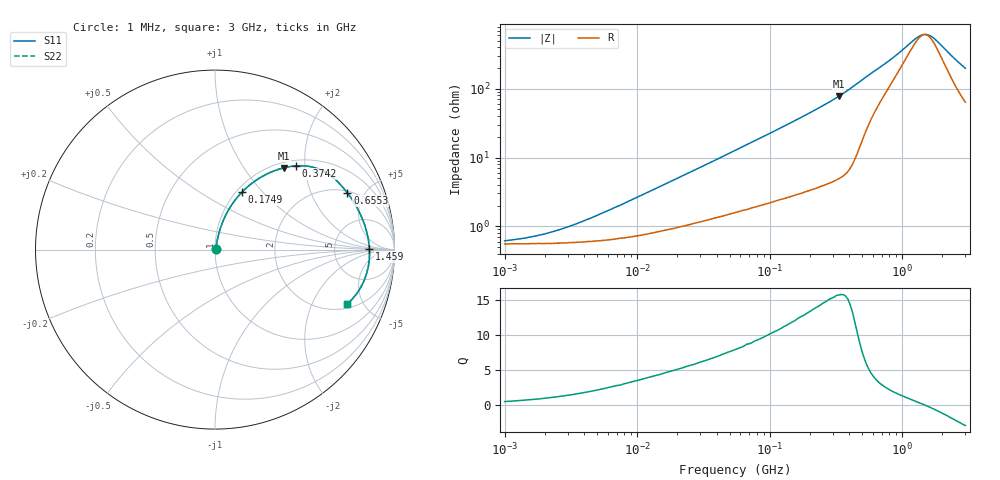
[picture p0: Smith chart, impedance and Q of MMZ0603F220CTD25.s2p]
! S-parameter Generated by TDK Corporation
! Copyright(C) 2018 TDK Corporation.
! All Rights Reserved.
! TDK P/N: MMZ0603F220CTD25 (Chip Bead)
! Property: |Z|=22¶ at 100MHz
! Size(LxWxT): 0.6x0.3x0.3mm, 0.024x0.012x0.012inches
! Model Type: s2p (Touchstone File Format Version 1.0)
! Frequency: DC=Yes Start=1MHz Stop=3000MHz 202points Log-sweep
! Model Generated on Aug. 6, 2018
! Port Assignments:
!  1 ---@@@--- 2
! Applicable Conditions:
!  Temperature = 25 degC
!  DC Bias Current = 0 A
!  Small Signal Operation
! Terms and conditions regarding TDK Simulation Models
! (1)This simulation model is being provided solely for informational purposes. Please refer to the specifications of the products in terms of detailed characteristics of such products.
! (2)In no event shall TDK Corporation of any of its subsidiaries be liable for any loss or damage arising, directly or indirectly,
!  From any information contained in this simulation model, including, but not limited to loss or damages arising from any inaccuracies, omissions or errors in connection with such information.
! (3)Any and all copyrights on this simulation model are owned by TDK Corporation.
!  Duplication or redistribution of this simulation model without prior written permission from TDK Corporation is prohibited.
! (4)This simulation model is subject to any modification or change without any prior notice.
! (5)Neither TDK Corporation nor any of its subsidiaries shall make any warranty, express or implied,
!  Including but not limited to the correctness, implied warranties of merchantability and fitness for a particular purpose with respect to this simulation models.
! (6)The use of this simulation model shall be deemed to have consented to the terms and conditions hereof.
# Hz S MA R 50
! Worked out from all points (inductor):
!   201 points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, 1 MHz to 3 GHz, reference 50 ohm
!   read as one part in series: L = 40.4 nH near 8.018 MHz
!   highest Q = 15.8 at 331.8 MHz (marker M1), where L = 37.1 nH
!   self-resonance near 1.473 GHz
!   S11 on the Smith chart (normalised r, x): 1 MHz: 1.01, +0.01; 174.9 MHz: 1.06, +0.77; 374.2 MHz: 1.12, +1.80; 655.3 MHz: 2.11, +3.75; 1.459 GHz: 13, +0; 3 GHz: 2.27, -3.76
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1000000  0.006099 25.4  0.9945 -0.2  0.9945 -0.2  0.006099 25.4
1974946  0.007628 42.7  0.9944 -0.3  0.9944 -0.3  0.007628 42.7
3900413  0.01176 59.5  0.9941 -0.6  0.9941 -0.6  0.01176 59.5
1.461624e7  0.03693 75.0  0.9911 -2.1  0.9911 -2.1  0.03693 75.0
3.00453e7  0.07113 76.7  0.9861 -4.0  0.9861 -4.0  0.07113 76.7
5.477226e7  0.1234 75.8  0.977 -7.0  0.977 -7.0  0.1234 75.8
1.081723e8  0.2298 71.3  0.9517 -13.2  0.9517 -13.2  0.2298 71.3
1.748812e8  0.3522 64.9  0.9087 -20.6  0.9087 -20.6  0.3522 64.9
2.136344e8  0.4182 61.2  0.8785 -24.6  0.8785 -24.6  0.4182 61.2
2.716345e8  0.5091 55.6  0.8274 -30.5  0.8274 -30.5  0.5091 55.6
3.318279e8  0.5944 50.0  0.7674 -36.4  0.7674 -36.4  0.5944 50.0
3.741707e8  0.6492 46.0  0.7203 -40.4  0.7203 -40.4  0.6492 46.0
4.570858e8  0.733 37.7  0.6142 -46.9  0.6142 -46.9  0.733 37.7
5.364635e8  0.7737 30.6  0.5169 -49.7  0.5169 -49.7  0.7737 30.6
6.553423e8  0.8027 23.2  0.4104 -50.3  0.4104 -50.3  0.8027 23.2
8.005644e8  0.8238 16.9  0.3192 -48.5  0.3192 -48.5  0.8238 16.9
1.294266e9  0.8566 3.6  0.1547 -20.3  0.1547 -20.3  0.8566 3.6
1.45942e9  0.8604 0.3  0.1397 -1.6  0.1397 -1.6  0.8604 0.3
1.581072e9  0.8613 -2.0  0.1424 12.1  0.1424 12.1  0.8613 -2.0
1.712864e9  0.861 -4.3  0.1557 24.7  0.1557 24.7  0.861 -4.3
2.266846e9  0.8445 -13.0  0.2591 46.9  0.2591 46.9  0.8445 -13.0
3e9  0.7962 -22.3  0.4013 49.0  0.4013 49.0  0.7962 -22.3
